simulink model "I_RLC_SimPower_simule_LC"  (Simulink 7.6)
settings: Solver=ode15s  StartTime=0.0  StopTime=0.14  RelTol=1e-3
PreLoadFcn:
  | clc
InitFcn:
  | R=1;     % 1 Ohm
  | L=0.01; % 10 mF
  | C=1e-3; % 1 mH
StopFcn:
  | close all
  | load I_RLC_SimPower.mat
  | plot(x(1,:),x(2,:))
  | hold on
  | plot(x(1,:),x(3,:))
  | plot(x(1,:),x(4,:))
  | %axis([0 0.14 -0.2 2.2])
  | grid
  | title('Courant dans le circuit RLC, tension aux bornes de C et échelon d''entrée')
  | ylabel('Circuit RLC - Simulation de la capacité et de l''inductance')
  | xlabel('temps')
libraries: powerlib x11

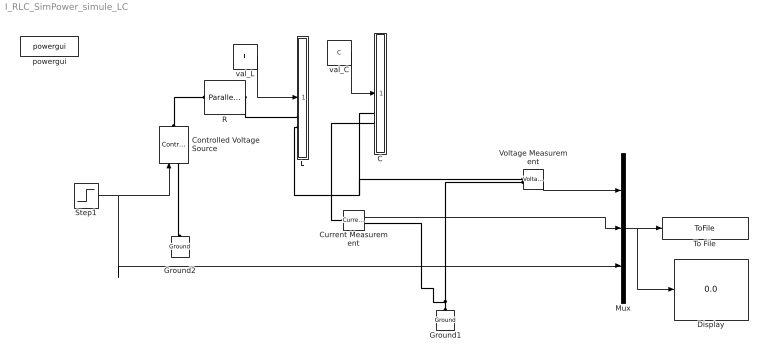
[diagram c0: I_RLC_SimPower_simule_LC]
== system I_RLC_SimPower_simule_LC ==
  C : Subsystem  mask{C=C}
      mask prompts: C "Capacite"
  Controlled Voltage Source : powerlib/Electrical Sources/Controlled Voltage Source  DialogController=POWERSYS.PowerSysDialog  SystemSampleTime=-1  Initialize=on  Source_Type=AC  Amplitude=0  Phase=0  Frequency=0  Measurements=None
  Current Measurement : powerlib/Measurements/Current Measurement  DialogController=POWERSYS.PowerSysDialog  SystemSampleTime=-1  PhasorSimulation=off  OutputType=Complex  PSBequivalent=0
  Display : Display
  Ground1 : powerlib/Elements/Ground  DialogController=POWERSYS.PowerSysDialog  PhysicalDomain=powersysdomain  SubClassName=unknown  LeftPortType=p1  RightPortType=p1  LConnTagsString=a
  Ground2 : powerlib/Elements/Ground  DialogController=POWERSYS.PowerSysDialog  PhysicalDomain=powersysdomain  SubClassName=unknown  LeftPortType=p1  RightPortType=p1  LConnTagsString=a
  L : Subsystem  mask{L=L}
      mask prompts: L "Inductance"
  Mux : Mux  Inputs=3
  R : powerlib/Elements/Parallel RLC Branch  DialogController=POWERSYS.PowerSysDialog  PhysicalDomain=powersysdomain  SubClassName=unknown  LeftPortType=p1  RightPortType=p1  LConnTagsString=a  RConnTagsString=__new0  BranchType=R  Resistance=2*R  Inductance=10e-03  SetiL0=off  InitialCurrent=0  Capacitance=[]  Setx0=off  InitialVoltage=0  Measurements=None
  Step1 : Step  Time=0.02  SampleTime=0
  To File : ToFile  Filename=I_RLC_SimPower  MatrixName=x
  Voltage Measurement : powerlib/Measurements/Voltage Measurement  DialogController=POWERSYS.PowerSysDialog  SystemSampleTime=-1  PhasorSimulation=off  OutputType=Complex  PSBequivalent=0
  powergui : powerlib/powergui  SystemSampleTime=-1  SimulationMode=Continuous  SampleTime=0  frequency=60  SPID=off  DisableSnubberDevices=off  DisableRonSwitches=off  DisableVfSwitches=off  SwTol=0  Interpol=off  frequencyindice=0  echomessages=off  HookPort=off  DisplayEquations=off  FunctionMessages=off  EnableUseOfTLC=off  x0status=blocks  RestoreLinks=warning  ResistiveCurrentMeasurement=off  Frange=[0:2:500]  Ylog=off  Xlog=on  ShowGrid=off  save=off  variable=ZData  ZoomFFT=on  StartTime=0.0  cycles=1  DisplayStyle=1  fundamental=60  FreqAxis=off  MaxFrequency=1000  frequencyindicesteady=60  RmsSteady=1  display=off  Ts=0  methode=off
  val_C : Constant  Value=C
  val_L : Constant  Value=L
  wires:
  Step1/1 -> Controlled Voltage Source/1, Mux/3
  Mux/1 -> To File/1, Display/1
  val_C/1 -> C/1(C)
  Current Measurement/1 -> Mux/2
  val_L/1 -> L/1(L)
  Voltage Measurement/1 -> Mux/1
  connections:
  Controlled Voltage Source/LConn1 -- Ground2/LConn1
  Ground1/LConn1 -- Voltage Measurement/LConn2 -- Current Measurement/RConn1
  Controlled Voltage Source/RConn1 -- R/RConn1
  R/LConn1 -- L/LConn1
  C/LConn1 -- L/LConn2 -- Voltage Measurement/LConn1
  Current Measurement/LConn1 -- C/LConn2

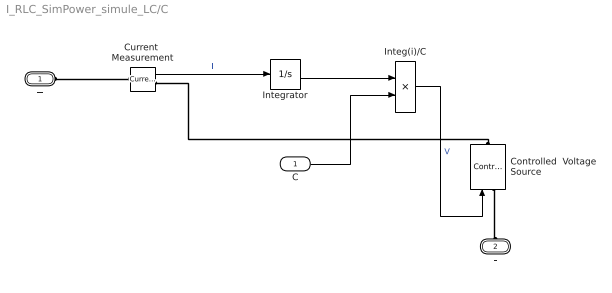
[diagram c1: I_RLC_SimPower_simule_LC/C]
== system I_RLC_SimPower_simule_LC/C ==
  C : Inport
  Controlled  Voltage Source : powerlib/Electrical Sources/Controlled Voltage Source  DialogController=POWERSYS.PowerSysDialog  SystemSampleTime=-1  Initialize=on  Source_Type=AC  Amplitude=0  Phase=0  Frequency=0  Measurements=None
  Current  Measurement : powerlib/Measurements/Current Measurement  DialogController=POWERSYS.PowerSysDialog  SystemSampleTime=-1  PhasorSimulation=off  OutputType=Complex  PSBequivalent=0
  Integ(i)/C : Product  Inputs=*/
  Integrator : Integrator
  + : PMIOPort  Port=1  Side=Left
  - : PMIOPort  Port=2  Side=Left
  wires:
  C/1 -> Integ(i)/C/2
  Current  Measurement/1 -> Integrator/1  "i"
  Integrator/1 -> Integ(i)/C/1
  Integ(i)/C/1 -> Controlled  Voltage Source/1  "V"
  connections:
  Current  Measurement/LConn1 -- +/RConn1
  Controlled  Voltage Source/LConn1 -- -/RConn1
  Controlled  Voltage Source/RConn1 -- Current  Measurement/RConn1

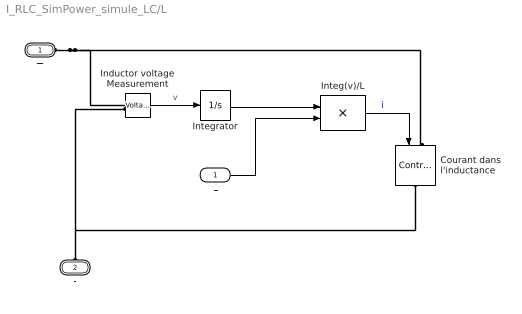
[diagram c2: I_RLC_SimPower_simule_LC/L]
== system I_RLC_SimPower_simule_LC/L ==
  L : Inport
  Courant dans  l'inductance : powerlib/Electrical Sources/Controlled Current Source  DialogController=POWERSYS.PowerSysDialog  SystemSampleTime=-1  Initialize=on  Source_Type=DC  Amplitude=0  Phase=0  Frequency=0  Measurements=None
  Inductor voltage Measurement : powerlib/Measurements/Voltage Measurement  DialogController=POWERSYS.PowerSysDialog  SystemSampleTime=-1  PhasorSimulation=off  OutputType=Magnitude  PSBequivalent=0
  Integ(v)/L : Product  Inputs=*/
  Integrator : Integrator
  + : PMIOPort  Port=1  Side=Left
  - : PMIOPort  Port=2  Side=Left
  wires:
  L/1 -> Integ(v)/L/2
  Inductor voltage Measurement/1 -> Integrator/1  "v"
  Integrator/1 -> Integ(v)/L/1
  Integ(v)/L/1 -> Courant dans  l'inductance/1  "i"
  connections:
  +/RConn1 -- Inductor voltage Measurement/LConn1 -- Courant dans  l'inductance/LConn1
  -/RConn1 -- Courant dans  l'inductance/RConn1 -- Inductor voltage Measurement/LConn2
